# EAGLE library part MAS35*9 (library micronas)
MAS® 35x9F MPEG Layer 2/3, AAC Audio Decoder, G.729 Annex A Codec Source: https://www.micronas.com .. mas35x9f_3ds.pdf
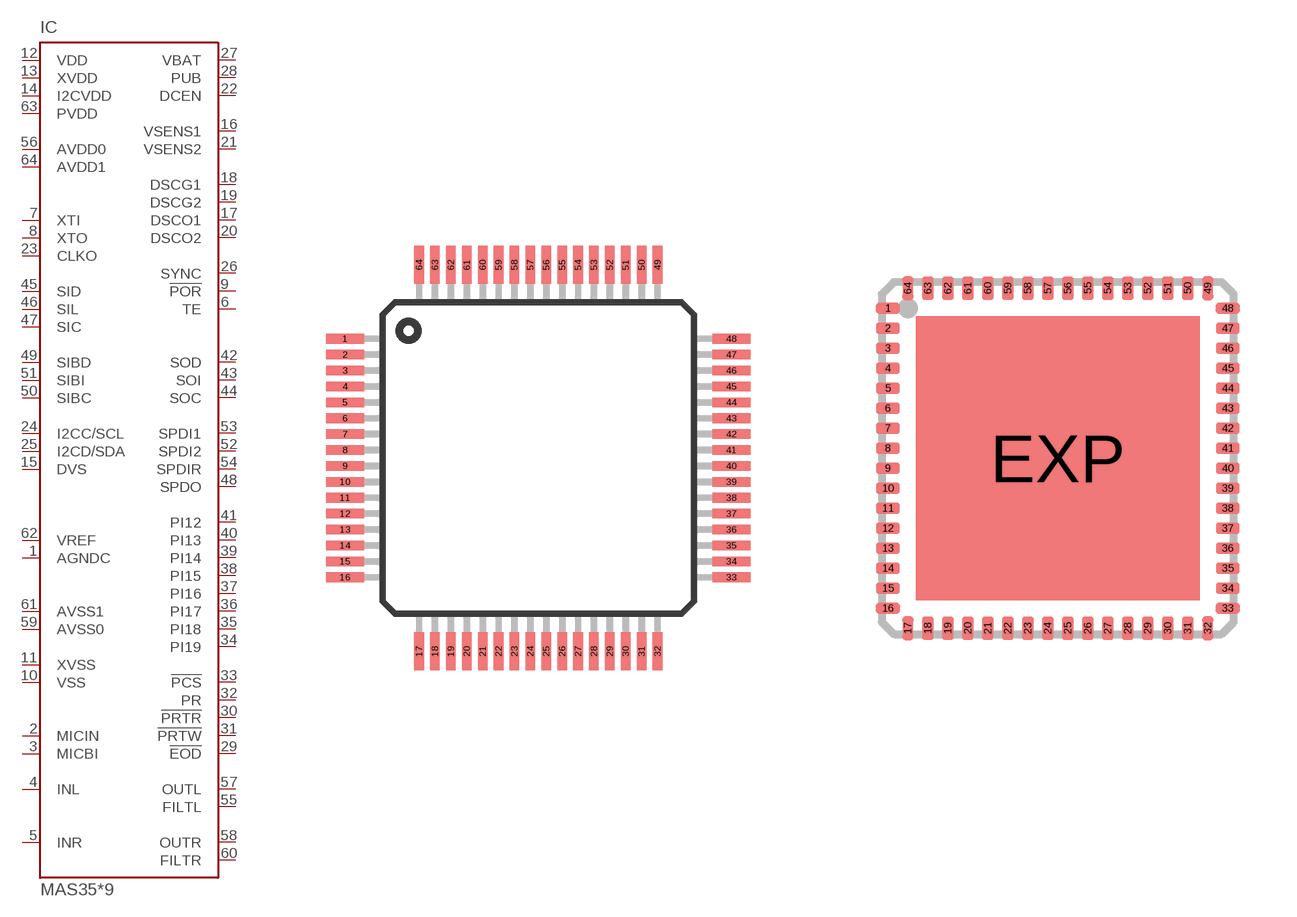
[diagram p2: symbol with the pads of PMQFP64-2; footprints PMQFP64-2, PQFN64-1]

Designator prefix IC

## MAS3519QI (OC_FARNELL: unknown; OC_NEWARK: unknown), MAS3529QI (OC_FARNELL: unknown; OC_NEWARK: unknown), MAS3539QI (OC_FARNELL: unknown; OC_NEWARK: unknown), MAS3549QI (OC_FARNELL: unknown; OC_NEWARK: unknown), MAS3559QI (OC_FARNELL: unknown; OC_NEWARK: unknown)  [PMQFP64-2]
1  AGNDC  pwr
2  MICIN  in
3  MICBI  in
4  INL  in
5  INR  in
6  TE  in
7  XTI  in
8  XTO  out
9  !POR  in
10  VSS  in
11  XVSS  in
12  VDD  in
13  XVDD  in
14  I2CVDD  in
15  DVS  in
16  VSENS1
17  DSCO1  pwr
18  DSCG1  pwr
19  DSCG2  pwr
20  DSCO2  pwr
21  VSENS2
22  DCEN  in
23  CLKO  out
24  I2CC/SCL
25  I2CD/SDA
26  SYNC  out
27  VBAT  in
28  PUB  out
29  !EOD  out
30  !PRTR  out
31  !PRTW  out
32  PR  in
33  !PCS  in
34  PI19
35  PI18
36  PI17
37  PI16
38  PI15
39  PI14
40  PI13
41  PI12
42  SOD  out
43  SOI  out
44  SOC  out
45  SID
46  SIL
47  SIC
48  SPDO  out
49  SIBD  in
50  SIBC  in
51  SIBI  in
52  SPDI2  in
53  SPDI1  in
54  SPDIR  in
55  FILTL  in
56  AVDD0  in
57  OUTL  out
58  OUTR  out
59  AVSS0  pwr
60  FILTR  in
61  AVSS1  pwr
62  VREF  in
63  PVDD  pwr
64  AVDD1  pwr

## MAS3519XK (OC_FARNELL: unknown; OC_NEWARK: unknown), MAS3529XK (OC_FARNELL: unknown; OC_NEWARK: unknown), MAS3539XK (OC_FARNELL: unknown; OC_NEWARK: unknown), MAS3549XK (OC_FARNELL: unknown; OC_NEWARK: unknown), MAS3559XK (OC_FARNELL: unknown; OC_NEWARK: unknown)  [PQFN64-1]
Pads as for PMQFP64-2

## MAS3519FH (OC_FARNELL: unknown; OC_NEWARK: unknown), MAS3529FH (OC_FARNELL: unknown; OC_NEWARK: unknown), MAS3539FH (OC_FARNELL: unknown; OC_NEWARK: unknown), MAS3549FH (OC_FARNELL: unknown; OC_NEWARK: unknown), MAS3559FH (OC_FARNELL: unknown; OC_NEWARK: unknown)  [PLQFP64-1]
Pads as for PMQFP64-2

## Footprint PMQFP64-2 (pad centres in mm)
Plastic Metric Quad Flat Package 64 leads, 10 × 10 × 2 mm³ Source: https://www.micronas.com .. mas35x9f_3ds.pdf
smd 1.2 x 0.3: 1 -6.075,3.75; 2 -6.075,3.25; 3 -6.075,2.75; 4 -6.075,2.25; 5 -6.075,1.75; 6 -6.075,1.25; 7 -6.075,0.75; 8 -6.075,0.25; 9 -6.075,-0.25; 10 -6.075,-0.75; 11 -6.075,-1.25; 12 -6.075,-1.75; 13 -6.075,-2.25; 14 -6.075,-2.75; 15 -6.075,-3.25; 16 -6.075,-3.75; 33 6.075,-3.75; 34 6.075,-3.25; 35 6.075,-2.75; 36 6.075,-2.25; 37 6.075,-1.75; 38 6.075,-1.25; 39 6.075,-0.75; 40 6.075,-0.25; 41 6.075,0.25; 42 6.075,0.75; 43 6.075,1.25; 44 6.075,1.75; 45 6.075,2.25; 46 6.075,2.75; 47 6.075,3.25; 48 6.075,3.75
smd 0.3 x 1.2: 17 -3.75,-6.075; 18 -3.25,-6.075; 19 -2.75,-6.075; 20 -2.25,-6.075; 21 -1.75,-6.075; 22 -1.25,-6.075; 23 -0.75,-6.075; 24 -0.25,-6.075; 25 0.25,-6.075; 26 0.75,-6.075; 27 1.25,-6.075; 28 1.75,-6.075; 29 2.25,-6.075; 30 2.75,-6.075; 31 3.25,-6.075; 32 3.75,-6.075; 49 3.75,6.075; 50 3.25,6.075; 51 2.75,6.075; 52 2.25,6.075; 53 1.75,6.075; 54 1.25,6.075; 55 0.75,6.075; 56 0.25,6.075; 57 -0.25,6.075; 58 -0.75,6.075; 59 -1.25,6.075; 60 -1.75,6.075; 61 -2.25,6.075; 62 -2.75,6.075; 63 -3.25,6.075; 64 -3.75,6.075

## Footprint PQFN64-1 (pad centres in mm)
Plastic Quad Flat Non-leaded package 64 pins, 9 × 9 × 0.85 mm³, 0.5 mm pitch Source: https://www.micronas.com .. mas35x9f_3ds.pdf
smd 0.6 x 0.28: 1 -4.25,3.75; 2 -4.25,3.25; 3 -4.25,2.75; 4 -4.25,2.25; 5 -4.25,1.75; 6 -4.25,1.25; 7 -4.25,0.75; 8 -4.25,0.25; 9 -4.25,-0.25; 10 -4.25,-0.75; 11 -4.25,-1.25; 12 -4.25,-1.75; 13 -4.25,-2.25; 14 -4.25,-2.75; 15 -4.25,-3.25; 16 -4.25,-3.75; 33 4.25,-3.75; 34 4.25,-3.25; 35 4.25,-2.75; 36 4.25,-2.25; 37 4.25,-1.75; 38 4.25,-1.25; 39 4.25,-0.75; 40 4.25,-0.25; 41 4.25,0.25; 42 4.25,0.75; 43 4.25,1.25; 44 4.25,1.75; 45 4.25,2.25; 46 4.25,2.75; 47 4.25,3.25; 48 4.25,3.75
smd 0.28 x 0.6: 17 -3.75,-4.25; 18 -3.25,-4.25; 19 -2.75,-4.25; 20 -2.25,-4.25; 21 -1.75,-4.25; 22 -1.25,-4.25; 23 -0.75,-4.25; 24 -0.25,-4.25; 25 0.25,-4.25; 26 0.75,-4.25; 27 1.25,-4.25; 28 1.75,-4.25; 29 2.25,-4.25; 30 2.75,-4.25; 31 3.25,-4.25; 32 3.75,-4.25; 49 3.75,4.25; 50 3.25,4.25; 51 2.75,4.25; 52 2.25,4.25; 53 1.75,4.25; 54 1.25,4.25; 55 0.75,4.25; 56 0.25,4.25; 57 -0.25,4.25; 58 -0.75,4.25; 59 -1.25,4.25; 60 -1.75,4.25; 61 -2.25,4.25; 62 -2.75,4.25; 63 -3.25,4.25; 64 -3.75,4.25
smd 7.1 x 7.1: EXP 0,0

## Footprint PLQFP64-1 (pad centres in mm)
Plastic Low Quad Flat Package 64 leads, 10 × 10 × 1.4 mm³ Source: https://www.micronas.com .. mas35x9f_3ds.pdf
smd 1 x 0.3: 1 -5.625,3.75; 2 -5.625,3.25; 3 -5.625,2.75; 4 -5.625,2.25; 5 -5.625,1.75; 6 -5.625,1.25; 7 -5.625,0.75; 8 -5.625,0.25; 9 -5.625,-0.25; 10 -5.625,-0.75; 11 -5.625,-1.25; 12 -5.625,-1.75; 13 -5.625,-2.25; 14 -5.625,-2.75; 15 -5.625,-3.25; 16 -5.625,-3.75; 33 5.625,-3.75; 34 5.625,-3.25; 35 5.625,-2.75; 36 5.625,-2.25; 37 5.625,-1.75; 38 5.625,-1.25; 39 5.625,-0.75; 40 5.625,-0.25; 41 5.625,0.25; 42 5.625,0.75; 43 5.625,1.25; 44 5.625,1.75; 45 5.625,2.25; 46 5.625,2.75; 47 5.625,3.25; 48 5.625,3.75
smd 0.3 x 1: 17 -3.75,-5.625; 18 -3.25,-5.625; 19 -2.75,-5.625; 20 -2.25,-5.625; 21 -1.75,-5.625; 22 -1.25,-5.625; 23 -0.75,-5.625; 24 -0.25,-5.625; 25 0.25,-5.625; 26 0.75,-5.625; 27 1.25,-5.625; 28 1.75,-5.625; 29 2.25,-5.625; 30 2.75,-5.625; 31 3.25,-5.625; 32 3.75,-5.625; 49 3.75,5.625; 50 3.25,5.625; 51 2.75,5.625; 52 2.25,5.625; 53 1.75,5.625; 54 1.25,5.625; 55 0.75,5.625; 56 0.25,5.625; 57 -0.25,5.625; 58 -0.75,5.625; 59 -1.25,5.625; 60 -1.75,5.625; 61 -2.25,5.625; 62 -2.75,5.625; 63 -3.25,5.625; 64 -3.75,5.625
